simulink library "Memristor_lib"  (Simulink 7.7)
settings: Solver=ode45  StartTime=0.0  StopTime=10.0  RelTol=1e-3
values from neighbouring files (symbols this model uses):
  v = M.*i    [MemristorToolbox.m]
undefined symbols (not defined in the file or in its folder): A, associative_memory_synapses, gcbh, HPmemristor, HPmemristor_BCM, HPmemristor_BCM_Generalized, HPmemristor_Biolek, HPmemristor_Joglekar, Ideal_memristor_1, m, Memristive_devices_example, Memristor, negresistor, nesl_callback, Novel_Memristor_1, Novel_Memristor_2, Ohm, s, V

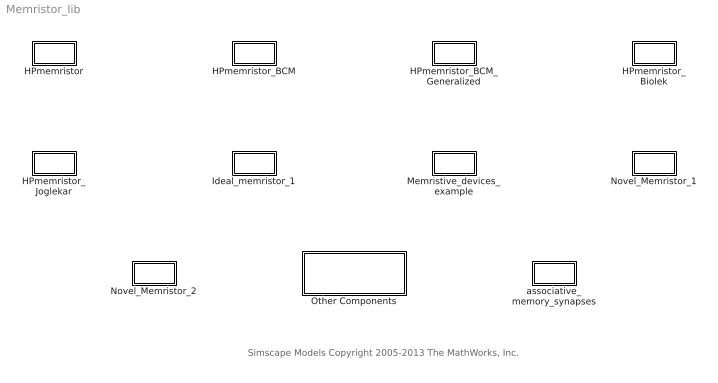
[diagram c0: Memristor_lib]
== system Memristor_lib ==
  note: Simscape Models Copyright 2005-2013 The MathWorks, Inc.
  HPmemristor : Subsystem  DialogController=NetworkEngine.DynNeDlgSource  LoadFcn=nesl_callback('LoadFcn',gcbh);  mask(HPmemristor){ComponentPath=Memristor.HPmemristor, ClassName=HPmemristor, SchemaVersion=1, R_off=100, R_off_unit=Ohm, R_on=2, R_on_unit=Ohm, u_v=1e-13, u_v_unit=m^2/s/V, D=1e-8, D_unit=m, w0=5e-9, w0_unit=m, i_Log=off, v_Log=off, w_Log=off, M_Log=off, LocalVarNames=\, LocalVarDescs=i\, LocalVarLogging=v\}
      mask init:
      | nesl_preinitmask (gcb);
  HPmemristor_BCM : Subsystem  DialogController=NetworkEngine.DynNeDlgSource  LoadFcn=nesl_callback('LoadFcn',gcbh);  mask(HPmemristor_BCM){ComponentPath=Memristor.HPmemristor_BCM, ClassName=HPmemristor_BCM, SchemaVersion=1, G_off=6e-5, G_off_unit=1/Ohm, G_on=0.0019, G_on_unit=1/Ohm, N=1, N_unit=1/Ohm, u_v=1e-14, u_v_unit=m^2/s/V, D=1e-8, D_unit=m, x0=0, x0_unit=Ohm, t0=1, t0_unit=s, i0=1, i0_unit=A, VT1=1, VT1_unit=V, VT0=1, VT0_unit=V, i_Log=off, v_Log=off, x_Log=off, F_Log=off, W_Log=off, LocalVarNames=\, LocalVarDescs=i\, LocalVarLogging=v\}
      mask init:
      | nesl_preinitmask (gcb);
  HPmemristor_BCM_Generalized : Subsystem  DialogController=NetworkEngine.DynNeDlgSource  LoadFcn=nesl_callback('LoadFcn',gcbh);  mask(HPmemristor_BCM_Generalized){ComponentPath=Memristor.HPmemristor_BCM_Generalized, ClassName=HPmemristor_BCM_Generalized, SchemaVersion=1, R_off=100, R_off_unit=Ohm, R_on=2, R_on_unit=Ohm, VTH1=0.2, VTH1_unit=V, VTH0=-0.2, VTH0_unit=V, VT1=0.2, VT1_unit=V, VT0=-0.2, VT0_unit=V, u_v=1e-13, u_v_unit=m^2/s/V, D=1e-8, D_unit=m, w0=5e-9, w0_unit=m, i_Log=off, v_Log=off, w_Log=off, F_Log=off, M_Log=off, LocalVarNames=\, LocalVarDescs=i\, LocalVarLogging=v\}
      mask init:
      | nesl_preinitmask (gcb);
  HPmemristor_Biolek : Subsystem  DialogController=NetworkEngine.DynNeDlgSource  LoadFcn=nesl_callback('LoadFcn',gcbh);  mask(HPmemristor_Biolek){ComponentPath=Memristor.HPmemristor_Biolek, ClassName=HPmemristor_Biolek, SchemaVersion=1, R_off=100, R_off_unit=Ohm, R_on=2, R_on_unit=Ohm, pp=1, pp_unit=m, u_v=1e-13, u_v_unit=m^2/s/V, D=1e-8, D_unit=m, w0=5e-9, w0_unit=m, i_Log=off, v_Log=off, w_Log=off, F_Log=off, M_Log=off, LocalVarNames=\, LocalVarDescs=i\, LocalVarLogging=v\}
      mask init:
      | nesl_preinitmask (gcb);
  HPmemristor_Joglekar : Subsystem  DialogController=NetworkEngine.DynNeDlgSource  LoadFcn=nesl_callback('LoadFcn',gcbh);  mask(HPmemristor_Joglekar){ComponentPath=Memristor.HPmemristor_Joglekar, ClassName=HPmemristor_Joglekar, SchemaVersion=1, R_off=100, R_off_unit=Ohm, R_on=2, R_on_unit=Ohm, pp=10, pp_unit=m, u_v=1e-13, u_v_unit=m^2/s/V, D=1e-8, D_unit=m, w0=5e-9, w0_unit=m, i_Log=off, v_Log=off, w_Log=off, F_Log=off, M_Log=off, LocalVarNames=\, LocalVarDescs=i\, LocalVarLogging=v\}
      mask init:
      | nesl_preinitmask (gcb);
  Ideal_memristor_1 : Subsystem  DialogController=NetworkEngine.DynNeDlgSource  LoadFcn=nesl_callback('LoadFcn',gcbh);  mask(Ideal_memristor_1){ComponentPath=Memristor.Ideal_memristor_1, ClassName=Ideal_memristor_1, SchemaVersion=1, M=1, M_unit=Ohm, x0=0.4, x0_unit=Ohm, i_Log=off, v_Log=off, x_Log=off, LocalVarNames=\, LocalVarDescs=i\, LocalVarLogging=v\}
      mask init:
      | nesl_preinitmask (gcb);
  Memristive_devices_example : Subsystem  DialogController=NetworkEngine.DynNeDlgSource  LoadFcn=nesl_callback('LoadFcn',gcbh);  mask(Memristive_devices_example){ComponentPath=Memristor.Memristive_devices_example, ClassName=Memristive_devices_example, SchemaVersion=1, x1_0=1, x1_0_unit=Ohm, x2_0=1, x2_0_unit=Ohm^0.50000, x3_0=1, x3_0_unit=Ohm, x4_0=1, x4_0_unit=Ohm^0.50000, x5_0=1, x5_0_unit=Ohm, i_Log=off, v_Log=off, x1_Log=off, x2_Log=off, x3_Log=off, x4_Log=off, x5_Log=off, M_Log=off, LocalVarNames=\, LocalVarDescs=i\, LocalVarLogging=v\}
      mask init:
      | nesl_preinitmask (gcb);
  Novel_Memristor_1 : Subsystem  DialogController=NetworkEngine.DynNeDlgSource  LoadFcn=nesl_callback('LoadFcn',gcbh);  mask(Novel_Memristor_1){ComponentPath=Memristor.Novel_Memristor_1, ClassName=Novel_Memristor_1, SchemaVersion=1, x0=0.4, x0_unit=Ohm, M=1, M_unit=Ohm/s, i_Log=off, v_Log=off, x_Log=off, LocalVarNames=\, LocalVarDescs=i\, LocalVarLogging=v\}
      mask init:
      | nesl_preinitmask (gcb);
  Novel_Memristor_2 : Subsystem  DialogController=NetworkEngine.DynNeDlgSource  LoadFcn=nesl_callback('LoadFcn',gcbh);  mask(Novel_Memristor_2){ComponentPath=Memristor.Novel_Memristor_2, ClassName=Novel_Memristor_2, SchemaVersion=1, x0=0.4, x0_unit=Ohm, M=10, M_unit=1/s/A, i_Log=off, v_Log=off, x_Log=off, LocalVarNames=\, LocalVarDescs=i\, LocalVarLogging=v\}
      mask init:
      | nesl_preinitmask (gcb);
  Other Components : Subsystem  Tag=simscape_sublibrary
  associative_memory_synapses : Subsystem  DialogController=NetworkEngine.DynNeDlgSource  LoadFcn=nesl_callback('LoadFcn',gcbh);  mask(associative_memory_synapses){ComponentPath=Memristor.associative_memory_synapses, ClassName=associative_memory_synapses, SchemaVersion=1, a=1.46e+5, a_unit=Ohm/s/V, B=1.46e+5, B_unit=Ohm/s/V, VT=4, VT_unit=V, R1=675, R1_unit=Ohm, R2=1e+4, R2_unit=Ohm, x0=1e+4, x0_unit=Ohm, i_Log=off, v_Log=off, x_Log=off, LocalVarNames=\, LocalVarDescs=i\, LocalVarLogging=v\}
      mask init:
      | nesl_preinitmask (gcb);

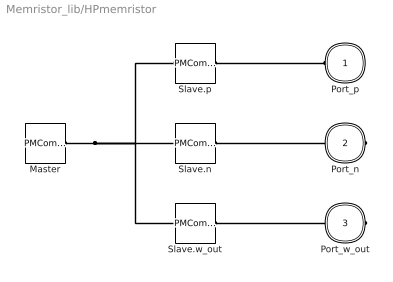
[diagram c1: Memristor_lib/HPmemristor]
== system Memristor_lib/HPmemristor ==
  Master : PMComponent  Tag=Memristor.HPmemristor  PhysicalDomain=network_engine_domain  SubClassName=master  LeftPortType=generic  RightPortType=generic  RConnTagsString=RConn1
  Slave.n : PMComponent  Tag=n  PhysicalDomain=network_engine_domain  SubClassName=terminal  LeftPortType=generic  RightPortType=foundation.electrical.electrical  LConnTagsString=LConn1  RConnTagsString=RConn1
  Slave.p : PMComponent  Tag=p  PhysicalDomain=network_engine_domain  SubClassName=terminal  LeftPortType=generic  RightPortType=foundation.electrical.electrical  LConnTagsString=LConn1  RConnTagsString=RConn1
  Slave.w_out : PMComponent  Tag=w_out  PhysicalDomain=network_engine_domain  SubClassName=output  LeftPortType=generic  RightPortType=output  LConnTagsString=LConn1  RConnTagsString=RConn1
  Port_p : PMIOPort  Tag=p  Port=1  Side=Left
  Port_n : PMIOPort  Tag=n  Port=2  Side=Right
  Port_w_out : PMIOPort  Tag=w_out  Port=3  Side=Right
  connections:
  Slave.p/RConn1 -- Port_p/RConn1
  Slave.p/LConn1 -- Slave.n/LConn1 -- Master/RConn1 -- Slave.w_out/LConn1
  Slave.n/RConn1 -- Port_n/RConn1
  Slave.w_out/RConn1 -- Port_w_out/RConn1

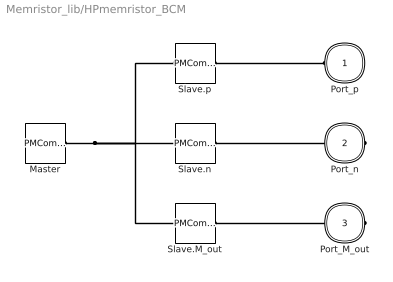
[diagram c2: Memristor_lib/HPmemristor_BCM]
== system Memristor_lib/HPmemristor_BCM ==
  Master : PMComponent  Tag=Memristor.HPmemristor_BCM  PhysicalDomain=network_engine_domain  SubClassName=master  LeftPortType=generic  RightPortType=generic  RConnTagsString=RConn1
  Slave.M_out : PMComponent  Tag=M_out  PhysicalDomain=network_engine_domain  SubClassName=output  LeftPortType=generic  RightPortType=output  LConnTagsString=LConn1  RConnTagsString=RConn1
  Slave.n : PMComponent  Tag=n  PhysicalDomain=network_engine_domain  SubClassName=terminal  LeftPortType=generic  RightPortType=foundation.electrical.electrical  LConnTagsString=LConn1  RConnTagsString=RConn1
  Slave.p : PMComponent  Tag=p  PhysicalDomain=network_engine_domain  SubClassName=terminal  LeftPortType=generic  RightPortType=foundation.electrical.electrical  LConnTagsString=LConn1  RConnTagsString=RConn1
  Port_p : PMIOPort  Tag=p  Port=1  Side=Left
  Port_n : PMIOPort  Tag=n  Port=2  Side=Right
  Port_M_out : PMIOPort  Tag=M_out  Port=3  Side=Right
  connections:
  Slave.p/RConn1 -- Port_p/RConn1
  Slave.p/LConn1 -- Slave.n/LConn1 -- Master/RConn1 -- Slave.M_out/LConn1
  Slave.n/RConn1 -- Port_n/RConn1
  Slave.M_out/RConn1 -- Port_M_out/RConn1

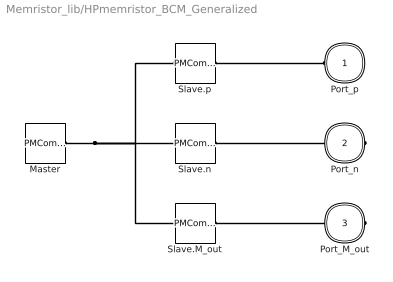
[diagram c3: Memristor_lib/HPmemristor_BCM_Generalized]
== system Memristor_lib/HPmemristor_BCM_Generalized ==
  Master : PMComponent  Tag=Memristor.HPmemristor_BCM_Generalized  PhysicalDomain=network_engine_domain  SubClassName=master  LeftPortType=generic  RightPortType=generic  RConnTagsString=RConn1
  Slave.M_out : PMComponent  Tag=M_out  PhysicalDomain=network_engine_domain  SubClassName=output  LeftPortType=generic  RightPortType=output  LConnTagsString=LConn1  RConnTagsString=RConn1
  Slave.n : PMComponent  Tag=n  PhysicalDomain=network_engine_domain  SubClassName=terminal  LeftPortType=generic  RightPortType=foundation.electrical.electrical  LConnTagsString=LConn1  RConnTagsString=RConn1
  Slave.p : PMComponent  Tag=p  PhysicalDomain=network_engine_domain  SubClassName=terminal  LeftPortType=generic  RightPortType=foundation.electrical.electrical  LConnTagsString=LConn1  RConnTagsString=RConn1
  Port_p : PMIOPort  Tag=p  Port=1  Side=Left
  Port_n : PMIOPort  Tag=n  Port=2  Side=Right
  Port_M_out : PMIOPort  Tag=M_out  Port=3  Side=Right
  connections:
  Slave.p/RConn1 -- Port_p/RConn1
  Slave.p/LConn1 -- Slave.n/LConn1 -- Master/RConn1 -- Slave.M_out/LConn1
  Slave.n/RConn1 -- Port_n/RConn1
  Slave.M_out/RConn1 -- Port_M_out/RConn1

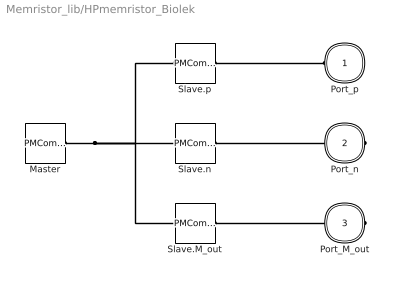
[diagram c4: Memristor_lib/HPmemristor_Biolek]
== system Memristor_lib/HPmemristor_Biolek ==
  Master : PMComponent  Tag=Memristor.HPmemristor_Biolek  PhysicalDomain=network_engine_domain  SubClassName=master  LeftPortType=generic  RightPortType=generic  RConnTagsString=RConn1
  Slave.M_out : PMComponent  Tag=M_out  PhysicalDomain=network_engine_domain  SubClassName=output  LeftPortType=generic  RightPortType=output  LConnTagsString=LConn1  RConnTagsString=RConn1
  Slave.n : PMComponent  Tag=n  PhysicalDomain=network_engine_domain  SubClassName=terminal  LeftPortType=generic  RightPortType=foundation.electrical.electrical  LConnTagsString=LConn1  RConnTagsString=RConn1
  Slave.p : PMComponent  Tag=p  PhysicalDomain=network_engine_domain  SubClassName=terminal  LeftPortType=generic  RightPortType=foundation.electrical.electrical  LConnTagsString=LConn1  RConnTagsString=RConn1
  Port_p : PMIOPort  Tag=p  Port=1  Side=Left
  Port_n : PMIOPort  Tag=n  Port=2  Side=Right
  Port_M_out : PMIOPort  Tag=M_out  Port=3  Side=Right
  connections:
  Slave.p/RConn1 -- Port_p/RConn1
  Slave.p/LConn1 -- Slave.n/LConn1 -- Master/RConn1 -- Slave.M_out/LConn1
  Slave.n/RConn1 -- Port_n/RConn1
  Slave.M_out/RConn1 -- Port_M_out/RConn1

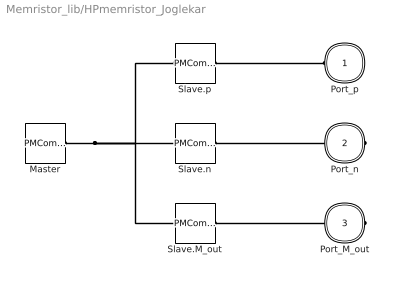
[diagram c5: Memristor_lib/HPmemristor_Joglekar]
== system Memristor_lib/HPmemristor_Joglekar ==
  Master : PMComponent  Tag=Memristor.HPmemristor_Joglekar  PhysicalDomain=network_engine_domain  SubClassName=master  LeftPortType=generic  RightPortType=generic  RConnTagsString=RConn1
  Slave.M_out : PMComponent  Tag=M_out  PhysicalDomain=network_engine_domain  SubClassName=output  LeftPortType=generic  RightPortType=output  LConnTagsString=LConn1  RConnTagsString=RConn1
  Slave.n : PMComponent  Tag=n  PhysicalDomain=network_engine_domain  SubClassName=terminal  LeftPortType=generic  RightPortType=foundation.electrical.electrical  LConnTagsString=LConn1  RConnTagsString=RConn1
  Slave.p : PMComponent  Tag=p  PhysicalDomain=network_engine_domain  SubClassName=terminal  LeftPortType=generic  RightPortType=foundation.electrical.electrical  LConnTagsString=LConn1  RConnTagsString=RConn1
  Port_p : PMIOPort  Tag=p  Port=1  Side=Left
  Port_n : PMIOPort  Tag=n  Port=2  Side=Right
  Port_M_out : PMIOPort  Tag=M_out  Port=3  Side=Right
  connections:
  Slave.p/RConn1 -- Port_p/RConn1
  Slave.p/LConn1 -- Slave.n/LConn1 -- Master/RConn1 -- Slave.M_out/LConn1
  Slave.n/RConn1 -- Port_n/RConn1
  Slave.M_out/RConn1 -- Port_M_out/RConn1

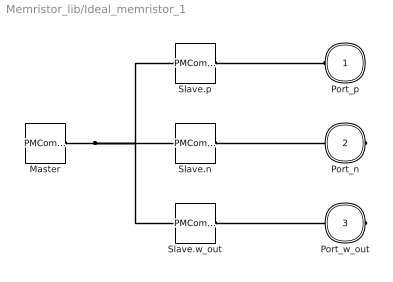
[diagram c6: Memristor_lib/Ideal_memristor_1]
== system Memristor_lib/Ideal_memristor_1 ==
  Master : PMComponent  Tag=Memristor.Ideal_memristor_1  PhysicalDomain=network_engine_domain  SubClassName=master  LeftPortType=generic  RightPortType=generic  RConnTagsString=RConn1
  Slave.n : PMComponent  Tag=n  PhysicalDomain=network_engine_domain  SubClassName=terminal  LeftPortType=generic  RightPortType=foundation.electrical.electrical  LConnTagsString=LConn1  RConnTagsString=RConn1
  Slave.p : PMComponent  Tag=p  PhysicalDomain=network_engine_domain  SubClassName=terminal  LeftPortType=generic  RightPortType=foundation.electrical.electrical  LConnTagsString=LConn1  RConnTagsString=RConn1
  Slave.w_out : PMComponent  Tag=w_out  PhysicalDomain=network_engine_domain  SubClassName=output  LeftPortType=generic  RightPortType=output  LConnTagsString=LConn1  RConnTagsString=RConn1
  Port_p : PMIOPort  Tag=p  Port=1  Side=Left
  Port_n : PMIOPort  Tag=n  Port=2  Side=Right
  Port_w_out : PMIOPort  Tag=w_out  Port=3  Side=Right
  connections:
  Slave.p/RConn1 -- Port_p/RConn1
  Slave.p/LConn1 -- Slave.n/LConn1 -- Master/RConn1 -- Slave.w_out/LConn1
  Slave.n/RConn1 -- Port_n/RConn1
  Slave.w_out/RConn1 -- Port_w_out/RConn1

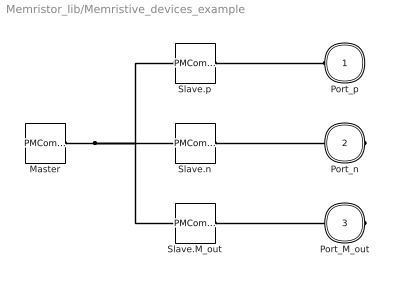
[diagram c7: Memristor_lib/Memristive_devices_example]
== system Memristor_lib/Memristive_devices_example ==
  Master : PMComponent  Tag=Memristor.Memristive_devices_example  PhysicalDomain=network_engine_domain  SubClassName=master  LeftPortType=generic  RightPortType=generic  RConnTagsString=RConn1
  Slave.M_out : PMComponent  Tag=M_out  PhysicalDomain=network_engine_domain  SubClassName=output  LeftPortType=generic  RightPortType=output  LConnTagsString=LConn1  RConnTagsString=RConn1
  Slave.n : PMComponent  Tag=n  PhysicalDomain=network_engine_domain  SubClassName=terminal  LeftPortType=generic  RightPortType=foundation.electrical.electrical  LConnTagsString=LConn1  RConnTagsString=RConn1
  Slave.p : PMComponent  Tag=p  PhysicalDomain=network_engine_domain  SubClassName=terminal  LeftPortType=generic  RightPortType=foundation.electrical.electrical  LConnTagsString=LConn1  RConnTagsString=RConn1
  Port_p : PMIOPort  Tag=p  Port=1  Side=Left
  Port_n : PMIOPort  Tag=n  Port=2  Side=Right
  Port_M_out : PMIOPort  Tag=M_out  Port=3  Side=Right
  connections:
  Slave.p/RConn1 -- Port_p/RConn1
  Slave.p/LConn1 -- Slave.n/LConn1 -- Master/RConn1 -- Slave.M_out/LConn1
  Slave.n/RConn1 -- Port_n/RConn1
  Slave.M_out/RConn1 -- Port_M_out/RConn1

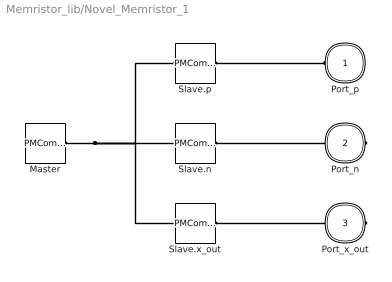
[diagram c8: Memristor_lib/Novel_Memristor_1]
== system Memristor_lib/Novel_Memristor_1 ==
  Master : PMComponent  Tag=Memristor.Novel_Memristor_1  PhysicalDomain=network_engine_domain  SubClassName=master  LeftPortType=generic  RightPortType=generic  RConnTagsString=RConn1
  Slave.n : PMComponent  Tag=n  PhysicalDomain=network_engine_domain  SubClassName=terminal  LeftPortType=generic  RightPortType=foundation.electrical.electrical  LConnTagsString=LConn1  RConnTagsString=RConn1
  Slave.p : PMComponent  Tag=p  PhysicalDomain=network_engine_domain  SubClassName=terminal  LeftPortType=generic  RightPortType=foundation.electrical.electrical  LConnTagsString=LConn1  RConnTagsString=RConn1
  Slave.x_out : PMComponent  Tag=x_out  PhysicalDomain=network_engine_domain  SubClassName=output  LeftPortType=generic  RightPortType=output  LConnTagsString=LConn1  RConnTagsString=RConn1
  Port_p : PMIOPort  Tag=p  Port=1  Side=Left
  Port_n : PMIOPort  Tag=n  Port=2  Side=Right
  Port_x_out : PMIOPort  Tag=x_out  Port=3  Side=Right
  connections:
  Slave.p/RConn1 -- Port_p/RConn1
  Slave.p/LConn1 -- Slave.n/LConn1 -- Master/RConn1 -- Slave.x_out/LConn1
  Slave.n/RConn1 -- Port_n/RConn1
  Slave.x_out/RConn1 -- Port_x_out/RConn1

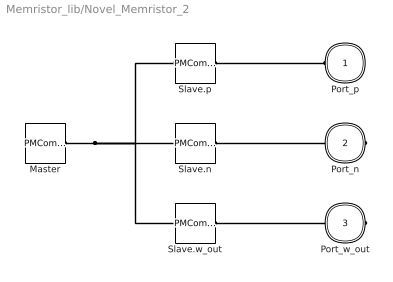
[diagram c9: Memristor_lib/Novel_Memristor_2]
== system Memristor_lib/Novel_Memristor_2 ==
  Master : PMComponent  Tag=Memristor.Novel_Memristor_2  PhysicalDomain=network_engine_domain  SubClassName=master  LeftPortType=generic  RightPortType=generic  RConnTagsString=RConn1
  Slave.n : PMComponent  Tag=n  PhysicalDomain=network_engine_domain  SubClassName=terminal  LeftPortType=generic  RightPortType=foundation.electrical.electrical  LConnTagsString=LConn1  RConnTagsString=RConn1
  Slave.p : PMComponent  Tag=p  PhysicalDomain=network_engine_domain  SubClassName=terminal  LeftPortType=generic  RightPortType=foundation.electrical.electrical  LConnTagsString=LConn1  RConnTagsString=RConn1
  Slave.w_out : PMComponent  Tag=w_out  PhysicalDomain=network_engine_domain  SubClassName=output  LeftPortType=generic  RightPortType=output  LConnTagsString=LConn1  RConnTagsString=RConn1
  Port_p : PMIOPort  Tag=p  Port=1  Side=Left
  Port_n : PMIOPort  Tag=n  Port=2  Side=Right
  Port_w_out : PMIOPort  Tag=w_out  Port=3  Side=Right
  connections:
  Slave.p/RConn1 -- Port_p/RConn1
  Slave.p/LConn1 -- Slave.n/LConn1 -- Master/RConn1 -- Slave.w_out/LConn1
  Slave.n/RConn1 -- Port_n/RConn1
  Slave.w_out/RConn1 -- Port_w_out/RConn1

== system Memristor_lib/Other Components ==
  note: Simscape Models Copyright 2005-2013 The MathWorks, Inc.
  Resistor : Subsystem  DialogController=NetworkEngine.DynNeDlgSource  LoadFcn=nesl_callback('LoadFcn',gcbh);  mask(Resistor){ComponentPath=Memristor.other_components.negresistor, ClassName=negresistor, SchemaVersion=1, R=1, R_unit=Ohm, i_Log=off, v_Log=off, LocalVarNames=\, LocalVarDescs=i\, LocalVarLogging=v}
      mask prompts: R "Resistance"
      mask help: The voltage-current (V-I) relationship for a linear resistor is V=I*R, where R is the constant resistance in ohms. The positive and negative terminals of the resistor are denoted by the + and - signs respectively. By convention, the voltage across the resistor is given by V(+)-V(-), and the sign of the current is positive when flowing through the device from the positive to the negative terminal. This convention ensures that the power absorbed by a resistor is always positive.
      mask init:
      | nesl_preinitmask (gcb);

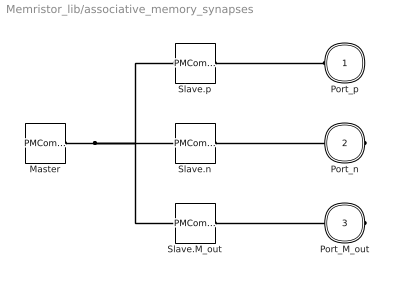
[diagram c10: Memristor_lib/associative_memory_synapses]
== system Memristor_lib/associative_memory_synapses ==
  Master : PMComponent  Tag=Memristor.associative_memory_synapses  PhysicalDomain=network_engine_domain  SubClassName=master  LeftPortType=generic  RightPortType=generic  RConnTagsString=RConn1
  Slave.M_out : PMComponent  Tag=M_out  PhysicalDomain=network_engine_domain  SubClassName=output  LeftPortType=generic  RightPortType=output  LConnTagsString=LConn1  RConnTagsString=RConn1
  Slave.n : PMComponent  Tag=n  PhysicalDomain=network_engine_domain  SubClassName=terminal  LeftPortType=generic  RightPortType=foundation.electrical.electrical  LConnTagsString=LConn1  RConnTagsString=RConn1
  Slave.p : PMComponent  Tag=p  PhysicalDomain=network_engine_domain  SubClassName=terminal  LeftPortType=generic  RightPortType=foundation.electrical.electrical  LConnTagsString=LConn1  RConnTagsString=RConn1
  Port_p : PMIOPort  Tag=p  Port=1  Side=Left
  Port_n : PMIOPort  Tag=n  Port=2  Side=Right
  Port_M_out : PMIOPort  Tag=M_out  Port=3  Side=Right
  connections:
  Slave.p/RConn1 -- Port_p/RConn1
  Slave.p/LConn1 -- Slave.n/LConn1 -- Master/RConn1 -- Slave.M_out/LConn1
  Slave.n/RConn1 -- Port_n/RConn1
  Slave.M_out/RConn1 -- Port_M_out/RConn1

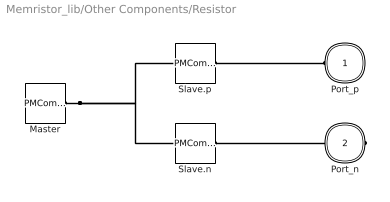
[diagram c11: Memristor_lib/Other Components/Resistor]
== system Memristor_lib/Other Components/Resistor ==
  Master : PMComponent  Tag=Memristor.other_components.negresistor  PhysicalDomain=network_engine_domain  SubClassName=master  LeftPortType=generic  RightPortType=generic  RConnTagsString=RConn1
  Slave.n : PMComponent  Tag=n  PhysicalDomain=network_engine_domain  SubClassName=terminal  LeftPortType=generic  RightPortType=foundation.electrical.electrical  LConnTagsString=LConn1  RConnTagsString=RConn1
  Slave.p : PMComponent  Tag=p  PhysicalDomain=network_engine_domain  SubClassName=terminal  LeftPortType=generic  RightPortType=foundation.electrical.electrical  LConnTagsString=LConn1  RConnTagsString=RConn1
  Port_p : PMIOPort  Tag=p  Port=1  Side=Left
  Port_n : PMIOPort  Tag=n  Port=2  Side=Right
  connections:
  Slave.p/RConn1 -- Port_p/RConn1
  Master/RConn1 -- Slave.p/LConn1 -- Slave.n/LConn1
  Slave.n/RConn1 -- Port_n/RConn1
